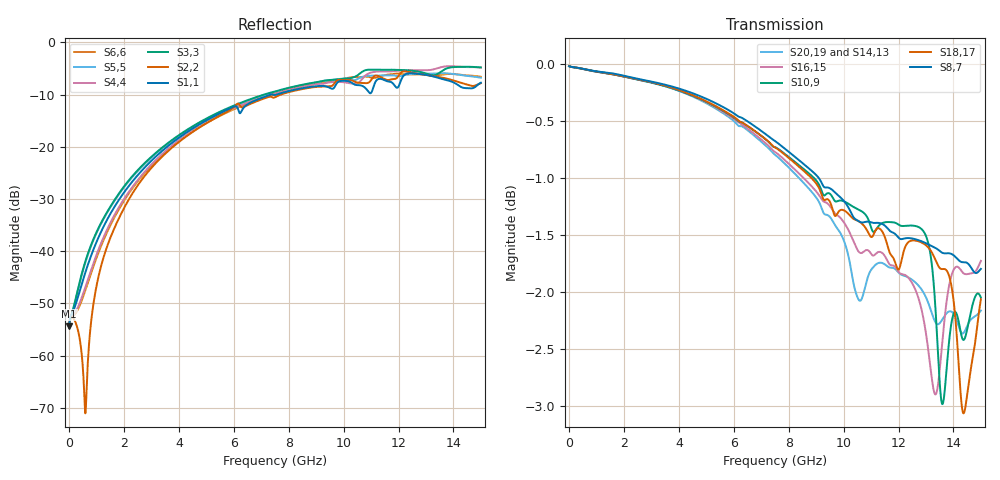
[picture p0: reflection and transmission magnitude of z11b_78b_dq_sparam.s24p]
![Disclaimer] This software code/ model/ data and all associated documentation, comments
!    or other information (collectively "Software") is provided
!    "AS IS" without warranty of any kind. MICRON TECHNOLOGY, INC.
!   ("MTI") EXPRESSLY DISCLAIMS ALL WARRANTIES EXPRESS OR IMPLIED,
!    INCLUDING BUT NOT LIMITED TO, NONINFRINGEMENT OF THIRD PARTY
!   RIGHTS, AND ANY IMPLIED WARRANTIES OF MERCHANTABILITY OR FITNESS
!    FOR ANY PARTICULAR PURPOSE. MTI DOES NOT WARRANT THAT THE
!    SOFTWARE WILL MEET YOUR REQUIREMENTS, OR THAT THE OPERATION OF
!    THE SOFTWARE WILL BE UNINTERRUPTED OR ERROR-FREE. FURTHERMORE,
!    MTI DOES NOT MAKE ANY REPRESENTATIONS REGARDING THE USE OR THE
!    RESULTS OF THE USE OF THE SOFTWARE IN TERMS OF ITS CORRECTNESS,
!    ACCURACY, RELIABILITY, OR OTHERWISE. THE ENTIRE RISK ARISING OUT
!    OF USE OR PERFORMANCE OF THE SOFTWARE REMAINS WITH YOU. IN NO
!    EVENT SHALL MTI, ITS AFFILIATED COMPANIES OR THEIR SUPPLIERS BE
!    LIABLE FOR ANY DIRECT, INDIRECT, CONSEQUENTIAL, INCIDENTAL, OR
!    SPECIAL DAMAGES (INCLUDING, WITHOUT LIMITATION, DAMAGES FOR LOSS
!    OF PROFITS, BUSINESS INTERRUPTION, OR LOSS OF INFORMATION)
!    ARISING OUT OF YOUR USE OF OR INABILITY TO USE THE SOFTWARE,
!    EVEN IF MTI HAS BEEN ADVISED OF THE POSSIBILITY OF SUCH DAMAGES.
!    Because some jurisdictions prohibit the exclusion or limitation
!    of liability for consequential or incidental damages, the above
!    limitation may not apply to you.
!    Copyright 2019 Micron Technology, Inc. All rights reserved.
! Single-ended  S-parameters
!NUMBER OF PORTS = 24
!  PORT#  PORT_NAME  NET_NAME
! PORT1:  DM#.BGA.VDDQ_VSS DM#
! PORT2:  DM#.Z11B_DIE.VDDQ_VSS DM#
! PORT3:  DQ0.BGA.VDDQ_VSS DQ0
! PORT4:  DQ0.Z11B_DIE.VDDQ_VSS DQ0
! PORT5:  DQ1.BGA.VDDQ_VSS DQ1
! PORT6:  DQ1.Z11B_DIE.VDDQ_VSS DQ1
! PORT7:  DQ2.BGA.VDDQ_VSS DQ2
! PORT8:  DQ2.Z11B_DIE.VDDQ_VSS DQ2
! PORT9:  DQ3.BGA.VDDQ_VSS DQ3
! PORT10:  DQ3.Z11B_DIE.VDDQ_VSS DQ3
! PORT11:  DQ4.BGA.VDDQ_VSS DQ4
! PORT12:  DQ4.Z11B_DIE.VDDQ_VSS DQ4
! PORT13:  DQ5.BGA.VDDQ_VSS DQ5
! PORT14:  DQ5.Z11B_DIE.VDDQ_VSS DQ5
! PORT15:  DQ6.BGA.VDDQ_VSS DQ6
! PORT16:  DQ6.Z11B_DIE.VDDQ_VSS DQ6
! PORT17:  DQ7.BGA.VDDQ_VSS DQ7
! PORT18:  DQ7.Z11B_DIE.VDDQ_VSS DQ7
! PORT19:  DQS-C.BGA.VDDQ_VSS DQS-C
! PORT20:  DQS-C.Z11B_DIE.VDDQ_VSS DQS-C
! PORT21:  DQS-T.BGA.VDDQ_VSS DQS-T
! PORT22:  DQS-T.Z11B_DIE.VDDQ_VSS DQS-T
! PORT23:  TDQS-C.BGA.VDDQ_VSS TDQS-C
! PORT24:  TDQS-C.Z11B_DIE.VDDQ_VSS TDQS-C
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# HZ S RI R 50
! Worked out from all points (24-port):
!   1701 points, 10 Hz to 15 GHz, reference 50 ohm
!   strongest paths, dB at 10 Hz, 2.25 GHz, 6.5 GHz, 10.75 GHz, 15 GHz:
!     S8,7: 0.0, -0.1, -0.5, -1.4, -1.8
!     S18,17: 0.0, -0.1, -0.5, -1.4, -2.1
!     S10,9: 0.0, -0.1, -0.5, -1.3, -2.0
!     S16,15: 0.0, -0.1, -0.6, -1.6, -1.7
!     S20,19: 0.0, -0.1, -0.6, -2.0, -2.2
!     S14,13: 0.0, -0.1, -0.6, -1.8, -2.5
!   lowest |S11| = -54.4 dB at 10 Hz (marker M1), VSWR 1.00, Z = 50.2 + j7.13e-08 ohm
!   |S11| at or under -10 dB: start of sweep to 7.334 GHz; 7.411 GHz to 7.563 GHz (152.2 MHz wide, 2.03 % of centre)
